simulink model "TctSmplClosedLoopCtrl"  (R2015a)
settings: Solver=ode3  SolverMode=SingleTasking  StartTime=0.0  StopTime=500  FixedStep=0.005  RelTol=1e-3

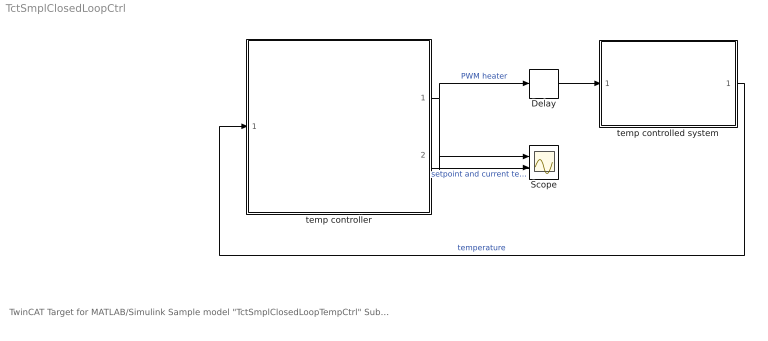
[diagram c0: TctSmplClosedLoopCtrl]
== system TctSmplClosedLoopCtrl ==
  note: TwinCAT Target for MATLAB/Simulink Sample model "TctSmplClosedLoopTempCtrl" Subjects: - Model Referencing - BusObjects
  Delay : Memory
  Scope : Scope  NumInputPorts=2
  temp controlled system : ModelReference  ModelNameDialog=TctSmplCtrlSysPT2  OverrideUsingVariant=varObject  ModelReferenceVersion=1.311  CopyOfModelName=TctSmplCtrlSysPT2
  temp controller : ModelReference  ModelNameDialog=TctSmplTempCtrl  ModelReferenceVersion=1.759  CopyOfModelName=TctSmplCtrlSysPT2
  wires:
  temp controlled system/1 -> temp controller/1  "temperature"
  Delay/1 -> temp controlled system/1
  temp controller/1 -> Delay/1, Scope/1  "PWM heater"
  temp controller/2 -> Scope/2  "setpoint and current temperature"
